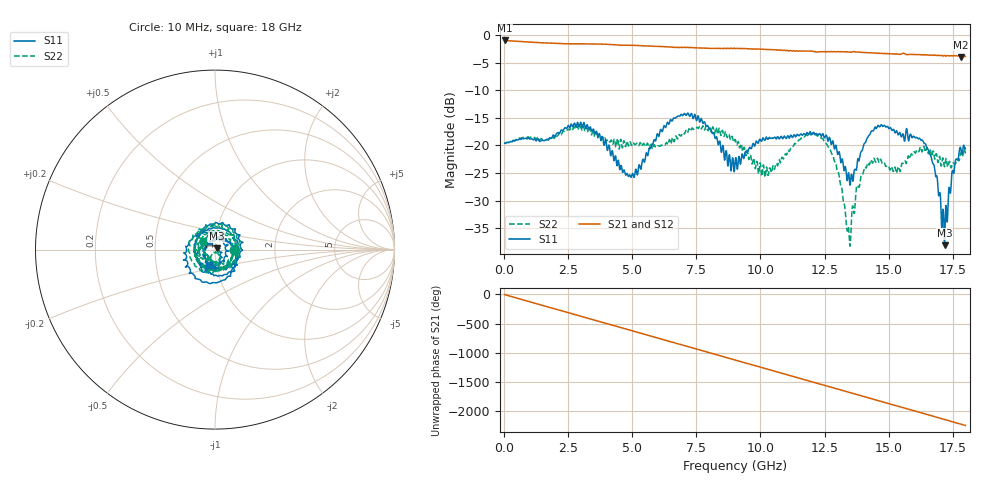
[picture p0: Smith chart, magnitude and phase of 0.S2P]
!Agilent Technologies,E5071C,MY46316741,A.11.02
!Date: Fri May 06 15:18:07 2022
!Data & Calibration Information:
!Freq	S11:SOLT2(ON)	S21:SOLT2(ON)	S12:SOLT2(ON)	S22:SOLT2(ON)
!PortZ  Port1:50+j0  Port2:50+j0
!Above PortZ is port z conversion or system Z0 setting when saving the data.
!When reading, reference impedance value at option line is always used.
# Hz S dB R 50
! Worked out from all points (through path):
!   1800 points, 10 MHz to 18 GHz, reference 50 ohm
!   highest |S21| = -0.99 dB at 10 MHz (marker M1); lowest = -4.0 dB at 17.84 GHz (marker M2)
!   group delay of S21, straight-line fit = 347 ps
!   lowest |S11| = -38.1 dB at 17.19 GHz (marker M3), VSWR 1.03, Z = 51 + j0.778 ohm
!   |S11| at or under -10 dB: start of sweep to end of sweep
!   |S22| runs from -38.2 to -16.5 dB; largest |S21 - S12| = 0.054
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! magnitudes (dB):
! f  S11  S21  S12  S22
! 10 MHz  -19.6  -1.0  -1.0  -19.6
! 3.01 GHz  -16.2  -1.6  -1.6  -17.0
! 3.77 GHz  -19.1  -1.7  -1.7  -18.7
! 4.89 GHz  -25.3  -1.9  -1.9  -19.5
! 6.01 GHz  -18.3  -2.1  -2.1  -20.0
! 7.37 GHz  -15.1  -2.3  -2.3  -17.1
! 9.01 GHz  -23.0  -2.5  -2.4  -18.9
! 10.24 GHz  -18.5  -2.6  -2.7  -23.9
! 12.01 GHz  -18.0  -2.9  -3.0  -17.9
! 12.87 GHz  -20.3  -3.0  -3.1  -22.5
! 13.12 GHz  -22.6  -3.0  -3.0  -27.0
! 13.44 GHz  -24.9  -3.1  -3.1  -35.1
! 13.81 GHz  -22.4  -3.1  -3.3  -27.4
! 14.12 GHz  -19.2  -3.2  -3.3  -24.1
! 15.01 GHz  -16.9  -3.4  -3.4  -23.8
! 16.4 GHz  -19.6  -3.6  -3.6  -20.5
! 16.82 GHz  -25.0  -3.7  -3.7  -22.3
! 17.12 GHz  -31.5  -3.8  -3.8  -22.3
! 17.19 GHz  -38.1  -3.7  -3.8  -23.9
! 17.55 GHz  -25.0  -3.7  -3.8  -23.3
! 17.84 GHz  -21.1  -4.0  -4.0  -21.5
! 18 GHz  -20.5  -3.9  -4.0  -21.6
